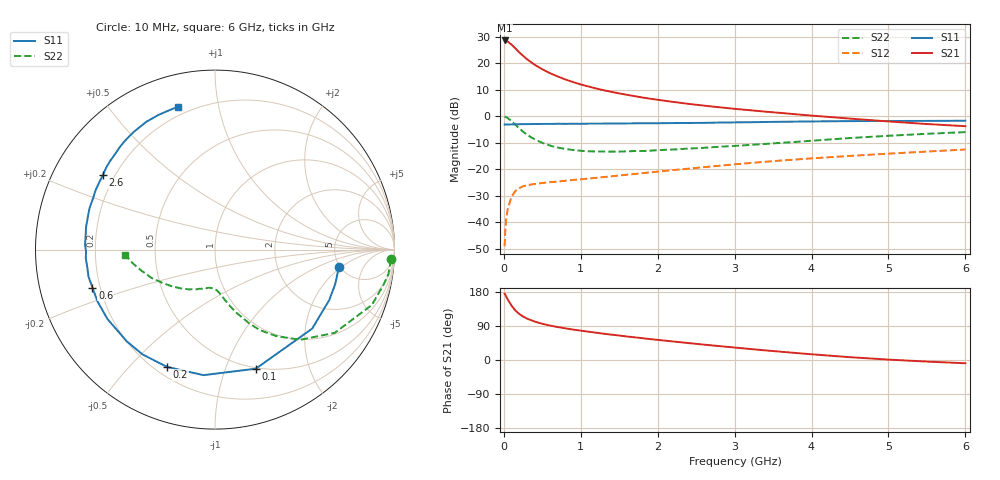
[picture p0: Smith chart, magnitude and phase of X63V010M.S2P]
! SIEMENS Small Signal Semiconductors
! BFP193W
! Si NPN RF Bipolar Junction Transistor in SOT343
! VCE = 3 V  IC = 10 mA
! Common Emitter S-Parameters:  April 1994
# GHz  S  MA  R  50
!  f  S11  S21  S12  S22
! GHz  MAG  ANG  MAG  ANG  MAG  ANG  MAG  ANG
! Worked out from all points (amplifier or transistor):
!   40 points, 10 MHz to 6 GHz, reference 50 ohm
!   highest |S21| = 28.6 dB at 10 MHz (marker M1)
!   |S21| within 3 dB of that: start of sweep to 150.5 MHz
!   unconditionally stable (mu >= 1): 1.296 GHz to 4.218 GHz
!   at 200 MHz: K = 0.22, MSG = 25.7 dB, |S12| = -27.2 dB
!   at 1.5 GHz: K = 1.06, MAG = 14.0 dB, |S12| = -22.4 dB
!   at 6 GHz: K = 0.92, MSG = 4.4 dB, |S12| = -12.6 dB
!   lowest NFmin = 1.30 dB at 450 MHz
!   S11 on the Smith chart (normalised r, x): 10 MHz: 4.89, -1.82; 100 MHz: 0.49, -1.28; 200 MHz: 0.25, -0.64; 600 MHz: 0.17, -0.15; 2.6 GHz: 0.16, +0.29; 6 GHz: 0.16, +0.76
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0.01  0.6969 -7.9  27.05 175.0  0.0035 88.1  0.9827 -3.2
0.02  0.697 -16.0  27.04 171.8  0.0074 82.2  0.9755 -8.1
0.03  0.6958 -23.9  26.76 167.8  0.0111 79.5  0.9591 -11.8
0.05  0.6979 -39.1  25.84 160.0  0.0176 72.1  0.927 -19.4
0.1  0.7014 -71.1  22.6 143.5  0.0303 58.4  0.8124 -34.8
0.15  0.7023 -95.2  19.18 130.7  0.0387 48.6  0.691 -46.7
0.2  0.7061 -112.2  16.18 121.6  0.0437 42.4  0.589 -54.8
0.25  0.71 -124.6  13.88 114.8  0.0475 37.8  0.5123 -61.0
0.3  0.7093 -133.9  11.98 109.4  0.0497 34.9  0.4481 -65.4
0.4  0.7131 -147.1  9.411 101.5  0.0525 31.8  0.3657 -71.8
0.5  0.7154 -156.1  7.708 95.5  0.0547 31.1  0.314 -76.2
0.6  0.7151 -162.8  6.5 90.9  0.0567 31.2  0.2791 -79.6
0.8  0.7184 -172.4  4.949 83.5  0.0604 32.7  0.2408 -84.5
1.1  0.7247 177.9  3.65 74.7  0.0664 35.9  0.2175 -90.9
1.3  0.7261 172.4  3.096 69.3  0.0709 38.2  0.215 -94.8
1.6  0.7315 165.4  2.54 62.0  0.0784 41.2  0.2168 -100.2
2.2  0.7428 153.7  1.867 48.9  0.0959 44.9  0.2349 -111.7
2.6  0.7495 146.5  1.587 40.6  0.109 45.9  0.2528 -119.5
3.2  0.7697 136.5  1.299 29.1  0.1304 45.6  0.2871 -131.1
4.5  0.8083 118.3  0.902 7.4  0.1778 41.1  0.3873 -156.0
5.5  0.8161 109.2  0.712 -4.2  0.2151 36.1  0.4654 -170.7
6  0.8221 104.6  0.648 -8.6  0.2347 33.7  0.5011 -176.5
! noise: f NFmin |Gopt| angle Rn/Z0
0.45  1.3  0.22  143  0.11
0.9  1.3  0.34  160  0.11
1.8  2.05  0.54  -153  0.14
